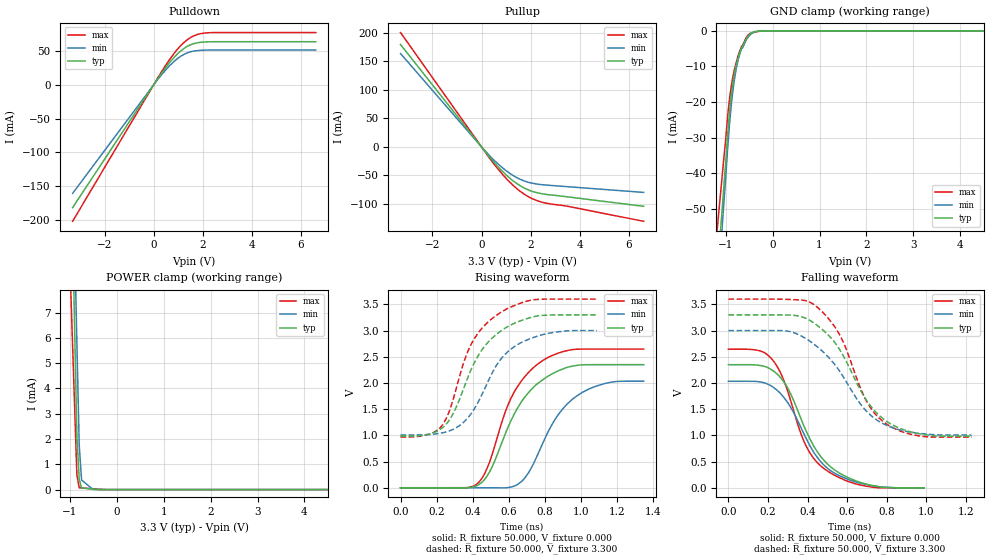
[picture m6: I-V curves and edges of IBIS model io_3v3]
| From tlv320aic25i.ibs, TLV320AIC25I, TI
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[Model]   io_3v3
Model_type I/O
Vinl=9.900E-01
Vinh=2.310E+00
Vref=0.000E+00
Rref=1.000E+06
Cref=2.000E-11
Vmeas=1.650E+00
C_comp   1.070E-12   1.070E-12   1.070E-12
[Voltage Range]   3.300E+00   3.000E+00   3.600E+00
[POWER Clamp Reference]   3.300E+00   3.000E+00   3.600E+00
[GND Clamp Reference]   0.000E+00   0.000E+00   0.000E+00
[Pullup Reference]   3.300E+00   3.000E+00   3.600E+00
[Pulldown Reference]   0.000E+00   0.000E+00   0.000E+00
[Temperature Range]   25   85   -40
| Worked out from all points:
|   slope of the pulldown table from 0 to 0.495 V, typ, clamps not added: 19.3 ohm
|   slope of the pullup table from 0 to 0.495 V, typ, clamps not added: 18.7 ohm
|   GND clamp passes 1 mA (typ) near -0.49 V on its own axis
|   POWER clamp passes 1 mA (typ) near -0.82 V on its own axis
|   rising waveform, R_fixture 50.000, V_fixture 0.000: 20-80 % time 210ps typ, 204ps min, 191ps max; typ from 0 V to 2.35 V
|   falling waveform, R_fixture 50.000, V_fixture 0.000: 20-80 % time 194ps typ, 191ps min, 166ps max; typ from 2.35 V to 0 V
|   rising waveform, R_fixture 50.000, V_fixture 3.300: 20-80 % time 207ps typ, 207ps min, 186ps max; typ from 0.985 V to 3.3 V
|   falling waveform, R_fixture 50.000, V_fixture 3.300: 20-80 % time 221ps typ, 237ps min, 187ps max; typ from 3.3 V to 0.985 V
[GND Clamp]
-3.3V     -442.3mA   -468.4mA   -354mA
-1.02V    -40.48mA   -44.95mA   -33.16mA
-940mV    -26.26mA   -30.01mA   -21.75mA
-900mV    -20.47mA   -23.54mA   -17.31mA
-860mV    -16mA      -18.37mA   -13.92mA
-780mV    -9.824mA   -11mA      -9.125mA
-720mV    -6.907mA   -7.44mA    -6.427mA
-660mV    -4.67mA    -4.99mA    -4.318mA
-560mV    -2.165mA   -2.517mA   -1.838mA
-460mV    -610.5uA   -873.5uA   -677.3uA
-240mV    0A         0A         0A
6.6V      0A         0A         0A
[POWER Clamp]
-3.3V     220.2mA    206.7mA    138.1mA
-1.1V     24.4mA     26.34mA    14.62mA
-850mV    2.148mA    5.848mA    588.7uA
-800mV    406.3uA    1.75mA     70.76uA
-750mV    62.13uA    376.4uA    64.33uA
-500mV    20.71uA    0A         32.16uA
-200mV    0A         0A         0A
6.6V      0A         0A         0A
[Pullup]
-3.3V     179.7mA    163.9mA    200.7mA
300mV     -16.69mA   -14.32mA   -18.17mA
860mV     -43.4mA    -36.94mA   -48.44mA
1.16V     -55.19mA   -46.65mA   -62.37mA
1.52V     -66.68mA   -55.73mA   -76.15mA
2.02V     -77.38mA   -63.23mA   -89.93mA
2.48V     -82.3mA    -66.34mA   -97.27mA
3.46V     -87.39mA   -69.63mA   -103.8mA
6.6V      -104.2mA   -79.83mA   -130.5mA
[Pulldown]
-3.3V     -181.7mA   -160.6mA   -201.9mA
200mV     10.99mA    9.561mA    12.37mA
620mV     31.68mA    27.24mA    36.04mA
860mV     41.73mA    35.54mA    47.88mA
1.08V     49.52mA    41.81mA    57.28mA
1.34V     56.37mA    46.84mA    65.93mA
1.52V     59.54mA    49.11mA    70.41mA
1.78V     62.24mA    50.68mA    74.51mA
2.16V     63.63mA    51.46mA    76.93mA
6.6V      63.85mA    51.62mA    77.36mA
[Rising Waveform]
R_fixture = 50.000
V_fixture = 0.000
V_fixture_min = 0.000
V_fixture_max = 0.000
|  time   V(typ)   V(min)   V(max)
0s        0V         0V         0V
430ps     50.06mV    0V         89.64mV
500ps     340mV      0V         544.3mV
580ps     1.014V     -1.498mV   1.431V
640ps     1.462V     44.42mV    1.879V
760ps     1.986V     620.7mV    2.356V
860ps     2.206V     1.316V     2.549V
950ps     2.318V     1.676V     2.634V
1.13ns    2.349V     1.985V     2.646V
1.35ns    2.349V     2.033V     2.646V
[Falling Waveform]
R_fixture = 50.000
V_fixture = 0.000
V_fixture_min = 0.000
V_fixture_max = 0.000
|  time   V(typ)   V(min)   V(max)
0s        2.349V     2.033V     2.646V
150ps     2.339V     2.026V     2.622V
220ps     2.249V     1.936V     2.455V
260ps     2.118V     1.812V     2.222V
300ps     1.902V     1.625V     1.841V
390ps     1.111V     966.8mV    821.5mV
490ps     497mV      409.5mV    349.6mV
570ps     263.9mV    217.8mV    179.6mV
690ps     78.94mV    68.51mV    37.9mV
990ps     0V         0V         0V
[Rising Waveform]
R_fixture = 50.000
V_fixture = 3.300
V_fixture_min = 3.000
V_fixture_max = 3.600
|  time   V(typ)   V(min)   V(max)
0s        984.8mV    1.008V     968.5mV
150ps     1.019V     1.012V     1.014V
230ps     1.137V     1.047V     1.186V
300ps     1.47V      1.128V     1.779V
390ps     2.24V      1.405V     2.724V
450ps     2.622V     1.765V     3.036V
530ps     2.921V     2.322V     3.285V
610ps     3.102V     2.638V     3.446V
730ps     3.255V     2.859V     3.583V
1.09ns    3.3V       3V         3.6V
[Falling Waveform]
R_fixture = 50.000
V_fixture = 3.300
V_fixture_min = 3.000
V_fixture_max = 3.600
|  time   V(typ)   V(min)   V(max)
0s        3.3V       3V         3.6V
300ps     3.297V     2.989V     3.595V
420ps     3.176V     2.776V     3.525V
490ps     2.97V      2.555V     3.298V
550ps     2.712V     2.293V     3.002V
590ps     2.457V     2.061V     2.7V
690ps     1.719V     1.496V     1.714V
780ps     1.326V     1.229V     1.273V
950ps     1.042V     1.046V     1.001V
1.23ns    984.8mV    1.008V     968.5mV
[Ramp]
dV/dt_r   1.409E+00/2.094E-10   1.221E+00/2.037E-10   1.588E+00/1.906E-10
dV/dt_f   1.389E+00/2.206E-10   1.195E+00/2.362E-10   1.579E+00/1.871E-10
R_load = 50
